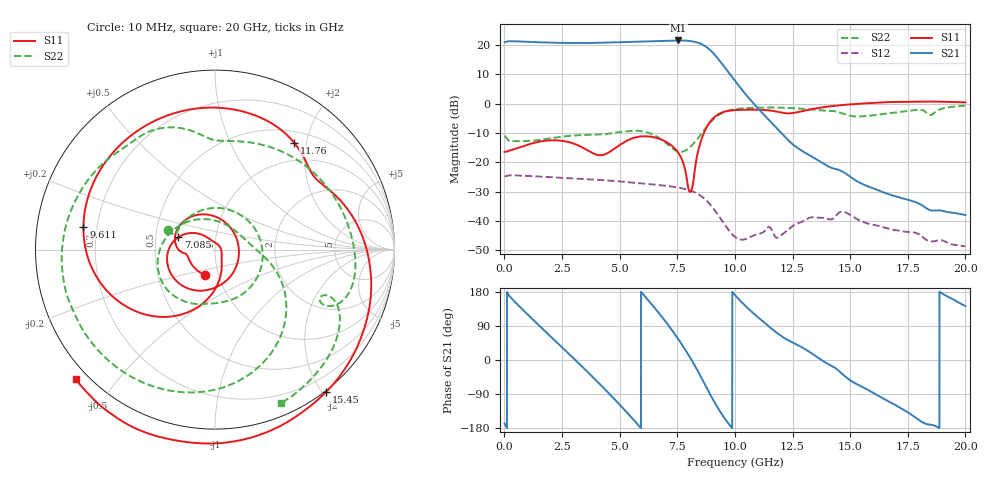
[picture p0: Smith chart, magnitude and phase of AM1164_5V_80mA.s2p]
!Agilent Technologies,E8364B,MY43040894,A.07.50.67
!Agilent E8364B: A.07.50.67
!Date: Wednesday, June 12, 2019 11:14:39
!Correction: S11(Full 2 Port(1,2))
!S21(Full 2 Port(1,2))
!S12(Full 2 Port(1,2))
!S22(Full 2 Port(1,2))
!S2P File: Measurements: S11, S21, S12, S22:
# Hz S  dB  R 50
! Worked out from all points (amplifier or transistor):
!   6401 points, 10 MHz to 20 GHz, reference 50 ohm
!   highest |S21| = 21.6 dB at 7.547 GHz (marker M1)
!   |S21| within 3 dB of that: start of sweep to 8.887 GHz
!   unconditionally stable (mu >= 1): start of sweep to 15.35 GHz
!   at 3.34 GHz: K = 1.11, MAG = 21.2 dB, |S12| = -25.6 dB
!   at 10.01 GHz: K = 5.42, MAG = 16.3 dB, |S12| = -45.4 dB
!   at 20 GHz: K = -166.46, MSG = 5.3 dB, |S12| = -48.5 dB
!   S11 on the Smith chart (normalised r, x): 10 MHz: 0.86, -0.25; 7.085 GHz: 0.65, +0.09; 9.611 GHz: 0.15, +0.09; 11.76 GHz: 0.68, +1.79; 15.45 GHz: -0.02, -2.05; 20 GHz: -0.03, -0.39
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1e7  -16.41 -111.8  20.96 -167.6  -24.81 13.1  -10.89 156.9
7.252672e8  -14.67 -175.3  21.21 137.0  -24.49 -36.2  -12.72 115.5
1.527991e9  -12.90 169.0  20.95 89.6  -24.81 -76.6  -12.33 47.6
2.524367e9  -12.66 134.1  20.74 32.1  -25.26 -126.3  -11.19 -22.3
3.342708e9  -14.72 89.4  20.71 -15.6  -25.61 -168.2  -10.68 -63.5
4.182912e9  -17.55 7.1  20.82 -66.1  -25.99 146.8  -10.45 -92.4
4.860698e9  -14.79 -68.4  20.95 -108.7  -26.37 109.2  -9.78 -111.7
5.835211e9  -11.21 -137.2  21.18 -173.6  -27.09 53.3  -9.24 -150.2
6.250628e9  -11.11 -160.1  21.27 157.2  -27.36 28.4  -9.90 -172.4
6.675416e9  -11.80 179.2  21.38 126.0  -27.68 1.7  -11.44 160.0
7.084586e9  -13.32 161.5  21.50 94.0  -28.03 -25.7  -13.88 125.4
7.546855e9  -16.73 140.7  21.58 54.8  -28.58 -59.4  -16.32 70.2
8.124691e9  -29.33 0.4  21.31 -0.5  -29.74 -107.5  -14.23 10.1
8.661922e9  -9.84 -104.9  19.87 -60.0  -32.21 -158.6  -9.01 -18.6
9.127314e9  -4.42 -150.0  16.67 -112.8  -36.34 158.7  -4.84 -47.8
9.611447e9  -2.56 170.0  11.89 -158.7  -41.74 129.6  -2.64 -78.5
1.0005e10  -2.16 143.5  7.80 171.4  -45.39 122.3  -1.87 -99.2
1.17635e10  -2.61 53.4  -7.88 74.4  -45.46 58.8  -1.28 -163.6
1.333771e10  -1.83 8.5  -17.96 17.2  -38.70 10.6  -1.94 147.8
1.545228e10  0.05 -52.0  -27.03 -68.8  -39.91 -91.0  -4.31 84.0
1.667042e10  0.56 -79.7  -30.83 -109.4  -42.58 -126.3  -3.26 43.0
2e10  0.49 -137.1  -37.91 142.7  -48.52 130.0  -0.62 -66.8
